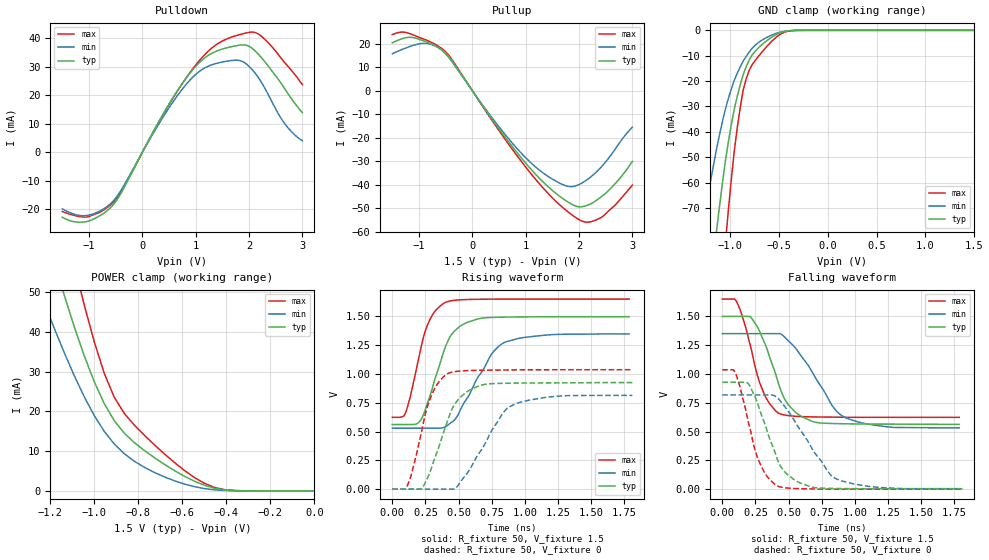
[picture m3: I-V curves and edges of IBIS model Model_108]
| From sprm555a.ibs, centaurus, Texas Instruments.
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| Model based on original model for BCSHTLTCSCDVPBFZ_SSGFV
|   Sub model SR10_12MA_10PER_1P5
[model]   Model_108
|[Description]  [1.5V-3-STATE-X-SLOW:12MA, IND, 10%]
|   Slow slew rate (SR[1:0] = "01"), 0.67 * RExt = 1.500 * Iout
|   (I[2:0] = "111"), 12mA nominal with Rext = 50R, ,Industrial
|   temperature range (-40C to 125C, 25C nominal),10% power supply
|   tolerance
|[Input Load]
|[Output Drive] SLOW:12MA
|Voltage   1.5V
|Mode   3-STATE
Model_type   3-state
Polarity   Non-Inverting
Enable   Active-Low
Cref =  15pF
Rref =  100.0000M
Vref =  0V
Vmeas =  0.75
C_comp   1.865048p   1.676829p   1.989968p
[Temperature Range]   25   125   -40
[Voltage Range]   1.5   1.35   1.65
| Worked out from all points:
|   slope of the pulldown table from 0 to 0.225 V, typ, clamps not added: 28.3 ohm
|   slope of the pullup table from 0 to 0.225 V, typ, clamps not added: 30.1 ohm
|   GND clamp passes 1 mA (typ) near -0.49 V on its own axis
|   POWER clamp passes 1 mA (typ) near -0.47 V on its own axis
|   rising waveform, R_fixture 50, V_fixture 1.5: 20-80 % time 163ps typ, 241ps min, 132ps max; typ from 0.561 V to 1.5 V
|   rising waveform, R_fixture 50, V_fixture 0: 20-80 % time 178ps typ, 250ps min, 140ps max; typ from 0 V to 0.925 V
|   falling waveform, R_fixture 50, V_fixture 1.5: 20-80 % time 185ps typ, 272ps min, 150ps max; typ from 1.5 V to 0.562 V
|   falling waveform, R_fixture 50, V_fixture 0: 20-80 % time 178ps typ, 278ps min, 145ps max; typ from 0.927 V to 0.004 V
[POWER_clamp]
-1.5V     126mA      88.79mA    168.7mA
-1.242V   69.8mA     49.45mA    94.34mA
-1.136V   49.16mA    34.72mA    67.51mA
-1.061V   36.35mA    25.4mA     50.03mA
-1.045V   33.92mA    23.63mA    46.66mA
-954.5mV  21.93mA    14.95mA    29.5mA
-909.1mV  17.64mA    11.79mA    23.52mA
-863.6mV  14.51mA    9.351mA    19.47mA
-772.7mV  10.16mA    5.94mA     13.99mA
-590.9mV  3.705mA    1.741mA    5.166mA
-454.5mV  710.5uA    279.1uA    892.1uA
0V        1.424nA    14.34nA    3.127nA
[Pulldown]
-1.5V     -22.72mA   -19.8mA    -20.72mA
-1.273V   -24.32mA   -21.69mA   -22.12mA
-1V       -24.04mA   -21.98mA   -22.46mA
-727.3mV  -21.41mA   -19.82mA   -20.23mA
-500mV    -17.33mA   -16.07mA   -16.65mA
681.8mV   22.29mA    20.49mA    22.2mA
1.045V    31.02mA    28.05mA    31.64mA
1.364V    35.28mA    31.06mA    37.46mA
1.818V    37.57mA    32.23mA    41.26mA
2.136V    35.16mA    27.23mA    41.87mA
2.636V    23.27mA    10.93mA    32.21mA
3V        13.9mA     4.109mA    23.75mA
[Pullup]
-1.5V     20.4mA     15.7mA     23.88mA
-1.136V   22.69mA    19.07mA    23.99mA
-863.6mV  20.8mA     20.11mA    21.55mA
-590.9mV  17.69mA    17.57mA    18.24mA
-409.1mV  13.64mA    13.19mA    14.12mA
909.1mV   -28.37mA   -26.41mA   -29.83mA
1.318V    -38.69mA   -34.9mA    -41.21mA
1.773V    -47.12mA   -40.66mA   -51.24mA
2.045V    -49.44mA   -39.45mA   -55.45mA
2.318V    -46.83mA   -34.79mA   -55.07mA
2.682V    -39.48mA   -24.74mA   -48.59mA
3V        -30.12mA   -15.56mA   -40.19mA
[GND_clamp]
-1.5V     -219.3mA   -131.6mA   -364.3mA
-1.288V   -134.4mA   -79.74mA   -225.6mA
-1.258V   -122.9mA   -72.77mA   -206.3mA
-1.136V   -79.27mA   -46.88mA   -132.4mA
-1.045V   -51.5mA    -31.06mA   -84.11mA
-1.015V   -44.02mA   -26.9mA    -70.91mA
-954.5mV  -31.01mA   -19.7mA    -47.55mA
-863.6mV  -17.48mA   -12.16mA   -23.55mA
-803mV    -11.81mA   -8.597mA   -15.85mA
-681.8mV  -5.986mA   -4.096mA   -9.026mA
-378.8mV  -126.2uA   -131.8uA   -179.7uA
1.5V      1.424nA    207.1nA    1.498nA
[Ramp]
dV/dt_f 0.56589432/0.18588572n 0.49496631/0.27330838n  0.6176321/0.15016945n
dV/dt_r 0.55954985/0.17888225n 0.49404507/0.25238762n 0.62420421/0.14056368n
R_load = 50
[Rising Waveform]
R_fixture = 50
V_fixture = 1.5
V_fixture_min = 1.35
V_fixture_max = 1.65
0s        560.9mV    529.1mV    623.9mV
98.3ps    560.9mV    529.1mV    657.5mV
215ps     601.4mV    529.1mV    1.22V
287.5ps   820.2mV    529.8mV    1.48V
396.1ps   1.22V      538.8mV    1.618V
453.7ps   1.353V     585.3mV    1.637V
535.4ps   1.431V     738.4mV    1.645V
751.3ps   1.491V     1.176V     1.649V
835.5ps   1.493V     1.267V     1.65V
1.787ns   1.497V     1.347V     1.65V
[Rising Waveform]
R_fixture = 50
V_fixture = 0
V_fixture_min = 0
V_fixture_max = 0
0s        0V         0V         0V
116.9ps   0V         0V         39.31mV
226ps     8.757mV    0V         528.4mV
308.4ps   230mV      0V         846.3mV
420.9ps   607.8mV    0V         1.005V
471ps     736.6mV    0V         1.02V
578.3ps   856.5mV    160.8mV    1.03V
897ps     919.9mV    722.5mV    1.035V
1.249ns   922.7mV    807.6mV    1.037V
1.811ns   925.5mV    814mV      1.037V
[Falling Waveform]
R_fixture = 50
V_fixture = 1.5
V_fixture_min = 1.35
V_fixture_max = 1.65
0s        1.499V     1.349V     1.649V
105.9ps   1.499V     1.349V     1.632V
216.9ps   1.489V     1.349V     1.222V
319.1ps   1.268V     1.349V     818.2mV
431ps     889.8mV    1.349V     656.1mV
491ps     742.6mV    1.296V     639.4mV
604.3ps   626.5mV    1.14V      629.3mV
918.8ps   567.3mV    626mV      623.9mV
1.29ns    564.1mV    535.9mV    623mV
1.787ns   562.2mV    532.1mV    622.9mV
[Falling Waveform]
R_fixture = 50
V_fixture = 0
V_fixture_min = 0
V_fixture_max = 0
0s        927mV      817.2mV    1.036V
99.2ps    927mV      817.2mV    1.01V
200.7ps   909.1mV    817.2mV    562.3mV
273.3ps   720.2mV    817.2mV    250.4mV
411.9ps   269.1mV    795.7mV    29.67mV
478.5ps   139.9mV    705.4mV    11.27mV
566.7ps   65.37mV    551.2mV    5.029mV
861.9ps   5.814mV    88.16mV    0V
1.183ns   3.936mV    14.85mV    0V
1.811ns   3.936mV    4.124mV    0V
